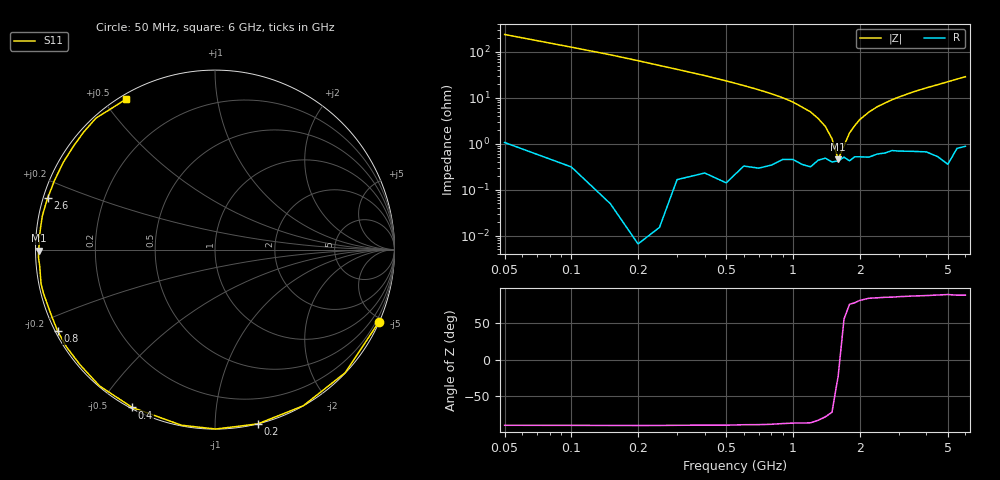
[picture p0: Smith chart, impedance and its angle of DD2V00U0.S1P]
! Infineon Technologies  Discrete & RF Semiconductors
! BBY58-02W
! Si Tuning Diode in SCD-80
! VR = 2 V
! S-Parameters:  June  2000
# GHz  S  MA  R  50
!  f  S11
! GHz  MAG  ANG
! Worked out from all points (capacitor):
!   34 points, 50 MHz to 6 GHz, reference 50 ohm
!   read as one part to ground: C = 12.6 pF near 50 MHz
!   lowest |Z| = 456 mohm at 1.6 GHz (marker M1)
!   series resonance near 1.619 GHz, so ESL is about 770 pH
!   S11 on the Smith chart (normalised r, x): 50 MHz: 0.02, -4.75; 200 MHz: 0.00, -1.28; 400 MHz: 0.00, -0.60; 800 MHz: 0.01, -0.24; 2.6 GHz: 0.01, +0.15; 6 GHz: 0.02, +0.57
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0.05  0.9982 -23.8
0.1  0.9983 -43.4
0.15  0.9995 -60.5
0.2  0.9999 -76.2
0.25  0.9997 -89.8
0.3  0.9961 -100.8
0.4  0.9933 -117.7
0.5  0.9954 -130.3
0.6  0.9886 -139.7
0.7  0.9893 -146.9
0.8  0.9872 -152.7
0.9  0.9827 -157.5
1.1  0.9862 -165.8
1.2  0.9877 -168.8
1.3  0.9828 -172.0
1.6  0.9833 -179.6
1.8  0.9833 176.2
2  0.9796 172.5
2.2  0.9801 169.0
2.4  0.9769 165.6
2.6  0.9759 162.7
3  0.9739 156.8
3.5  0.975 150.0
4  0.9764 143.8
4.5  0.982 138.1
5  0.9882 132.1
5.5  0.9752 126.2
6  0.974 120.5
